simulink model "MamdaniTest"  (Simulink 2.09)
settings: Solver=ode45  StartTime=0.0  StopTime=10  MaxStep=10  RelTol=1e-3  AbsTol=1e-3
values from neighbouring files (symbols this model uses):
  k_s = 1.1    [Mdata.m]    (also in Mdata25.m)
  tau = 1    [Mdata.m]    (also in Mdata25.m; VdataC.m = m/kv)
undefined symbols (not defined in the file or in its folder): sfunyst
libraries: fuzzy x1

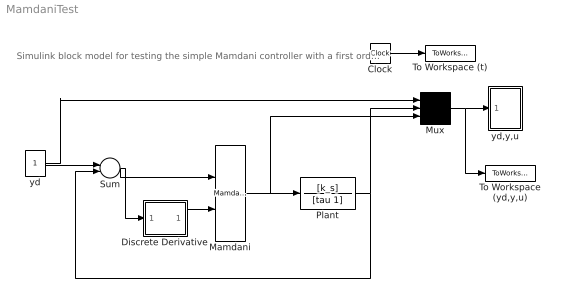
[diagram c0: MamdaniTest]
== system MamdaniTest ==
  note: Simulink block model for testing the simple Mamdani controller with a first order plan
  Clock : Clock
  Discrete Derivative : Subsystem
  Mamdani : fuzzy/Mamdani
  Mux : Mux  Inputs=3
  Plant : TransferFcn  Numerator=[k_s]  Denominator=[tau 1]
  Sum : Sum  Inputs=+-
  To Workspace (yd,y,u) : ToWorkspace  VariableName=yout  SampleTime=0
  To Workspace (t) : ToWorkspace  VariableName=t  SampleTime=0
  yd : Constant  Value=1
  yd,y,u : Subsystem  mask(Storage scope.){}
      mask help: Storage scope using MATLAB graph window. Enter plotting ranges and line type.
      mask init:
      | npts = @4; color = @5; ax = [0, @1, @2, @3]; dt=-1;
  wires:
  Mux/1 -> yd,y,u/1(x), To Workspace (yd,y,u)/1
  yd/1 -> Mux/1, Sum/1
  Mamdani/1 -> Plant/1, Mux/3
  Discrete Derivative/1(out_1) -> Mamdani/2
  Sum/1 -> Discrete Derivative/1(in_1), Mamdani/1
  Plant/1 -> Mux/2, Sum/2
  Clock/1 -> To Workspace (t)/1

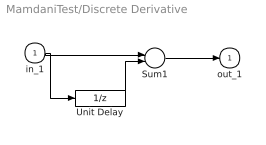
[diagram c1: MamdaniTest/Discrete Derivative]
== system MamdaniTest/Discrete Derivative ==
  in_1 : Inport  Port=1  PortWidth=-1  SampleTime=-1
  Sum1 : Sum  Inputs=+-
  Unit Delay : UnitDelay  X0=0  SampleTime=1
  out_1 : Outport  Port=1  InitialOutput=0
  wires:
  Unit Delay/1 -> Sum1/2
  Sum1/1 -> out_1/1
  in_1/1 -> Sum1/1, Unit Delay/1

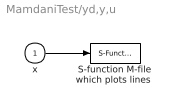
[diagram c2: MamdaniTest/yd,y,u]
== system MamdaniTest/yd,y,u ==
  x : Inport  Port=1  PortWidth=-1  SampleTime=-1
  "S-function M-file which plots lines " : S-Function  LoadFcn=sfunyst([],[],[],'LoadBlock')  FunctionName=sfunyst  Parameters=ax, color, npts, dt
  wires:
  x/1 -> "S-function M-file which plots lines "/1
